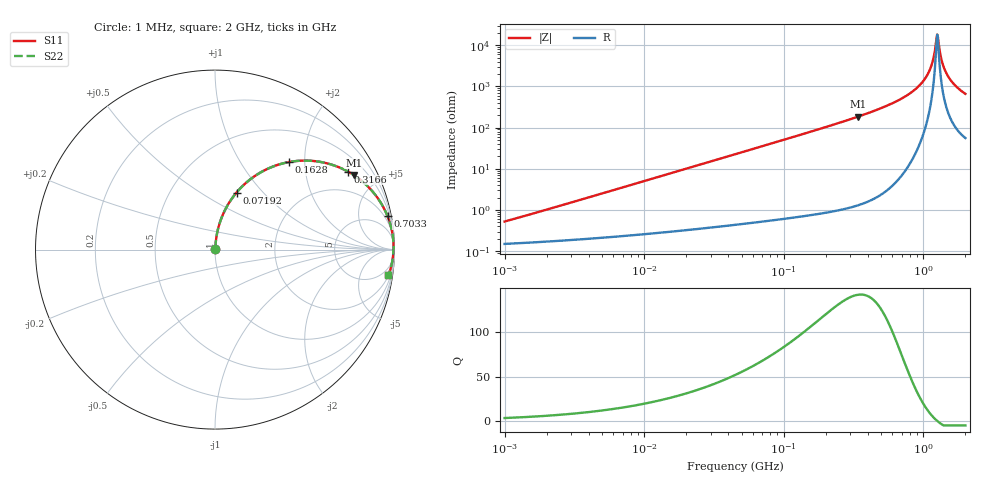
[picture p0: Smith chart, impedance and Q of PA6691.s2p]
# MHz S MA R 50
!Freq  MagS11  AngS11  MagS21  AngS21  MagS12  AngS12  MagS22  AngS22
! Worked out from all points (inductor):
!   801 points, 1 MHz to 2 GHz, reference 50 ohm
!   read as one part in series: L = 80 nH near 1.039 MHz
!   highest Q = 142 at 341.6 MHz (marker M1), where L = 86.4 nH
!   self-resonance near 1.256 GHz
!   S11 on the Smith chart (normalised r, x): 1 MHz: 1.00, +0.01; 71.92 MHz: 1.01, +0.73; 162.8 MHz: 1.02, +1.66; 316.6 MHz: 1.02, +3.40; 703.3 MHz: 1, +10; 2 GHz: 2, -13
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1  0.005238 73.1  0.9985 -0.3  0.9985 -0.3  0.005238 73.1
3.572091  0.01802 82.8  0.9979 -1.0  0.9979 -1.0  0.01802 82.8
12.63918  0.0633 83.9  0.9952 -3.6  0.9952 -3.6  0.0633 83.9
45.14829  0.2207 76.2  0.9711 -12.7  0.9711 -12.7  0.2207 76.2
71.91664  0.3394 69.3  0.9357 -19.8  0.9357 -19.8  0.3394 69.3
159.7488  0.6294 50.5  0.7712 -39.0  0.7712 -39.0  0.6294 50.5
162.8134  0.6369 49.9  0.7651 -39.6  0.7651 -39.6  0.6369 49.9
316.6141  0.8592 30.4  0.5057 -59.2  0.5057 -59.2  0.8592 30.4
341.6178  0.8775 28.3  0.4734 -61.3  0.4734 -61.3  0.8775 28.3
565.2411  0.9604 15.7  0.2698 -73.8  0.2698 -73.8  0.9604 15.7
703.2964  0.9791 11.0  0.1905 -78.2  0.1905 -78.2  0.9791 11.0
883.4242  0.9904 6.5  0.1132 -81.9  0.1132 -81.9  0.9904 6.5
1038.284  0.9942 3.5  0.06099 -82.8  0.06099 -82.8  0.9942 3.5
1141.771  0.9949 1.8  0.03106 -79.7  0.03106 -79.7  0.9949 1.8
1174.784  0.9949 1.2  0.02226 -76.2  0.02226 -76.2  0.9949 1.2
1220.29  0.9948 0.6  0.01104 -61.7  0.01104 -61.7  0.9948 0.6
1255.573  0.9946 0.0  0.005452 -8.6  0.005452 -8.6  0.9946 0.0
1291.876  0.9943 -0.5  0.009905 54.7  0.009905 54.7  0.9943 -0.5
1380.717  0.9932 -1.7  0.0297 76.0  0.0297 76.0  0.9932 -1.7
1489.756  0.9913 -3.0  0.05344 79.1  0.05344 79.1  0.9913 -3.0
1701.7  0.9862 -5.5  0.09566 79.0  0.09566 79.0  0.9862 -5.5
2000  0.9765 -8.5  0.1482 76.7  0.1482 76.7  0.9765 -8.5
